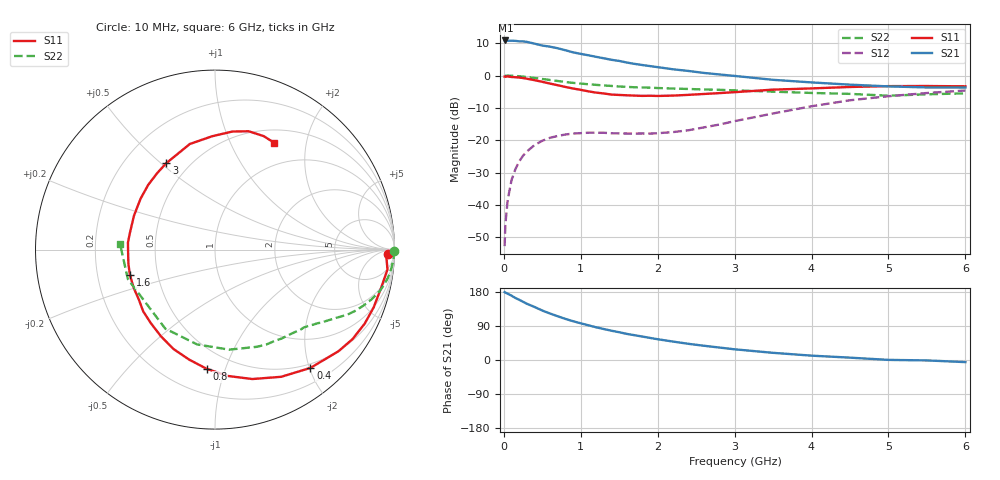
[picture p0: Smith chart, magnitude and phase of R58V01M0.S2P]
! SIEMENS Small Signal Semiconductors
! BFR183
! Si NPN RF Bipolar Junction Transistor in SOT23
! VCE = 8 V  IC = 1 mA
! Common Emitter S-Parameters:  May  1996
# GHz  S  MA  R  50
!  f  S11  S21  S12  S22
! GHz  MAG  ANG  MAG  ANG  MAG  ANG  MAG  ANG
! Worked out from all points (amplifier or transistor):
!   36 points, 10 MHz to 6 GHz, reference 50 ohm
!   highest |S21| = 10.8 dB at 20 MHz (marker M1)
!   |S21| within 3 dB of that: start of sweep to 796.1 MHz
!   unconditionally stable (mu >= 1): 1.684 GHz to 2.971 GHz
!   at 250 MHz: K = 0.15, MSG = 17.7 dB, |S12| = -24.8 dB
!   at 1.4 GHz: K = 0.85, MSG = 11.3 dB, |S12| = -17.8 dB
!   at 6 GHz: K = 0.95, MSG = 0.5 dB, |S12| = -4.6 dB
!   S11 on the Smith chart (normalised r, x): 10 MHz: 39, -23; 400 MHz: 0.43, -2.02; 800 MHz: 0.36, -0.86; 1.6 GHz: 0.34, -0.13; 3 GHz: 0.38, +0.52; 6 GHz: 0.66, +1.48
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0.01  0.9623 -1.3  3.439 179.3  0.0023 89.8  0.9985 -0.4
0.02  0.9561 -2.6  3.483 177.8  0.005 84.9  0.9919 -0.9
0.05  0.9673 -6.6  3.453 174.9  0.0119 83.9  0.997 -2.4
0.1  0.9493 -13.2  3.446 169.8  0.0242 82.0  0.9912 -4.8
0.15  0.9408 -20.0  3.433 163.7  0.0356 77.5  0.9842 -7.3
0.25  0.9144 -33.0  3.369 153.6  0.0576 70.2  0.9626 -11.7
0.3  0.8913 -39.4  3.314 148.3  0.067 67.0  0.9481 -13.9
0.4  0.8469 -51.1  3.106 139.9  0.0842 60.1  0.9157 -17.6
0.5  0.7989 -62.5  2.904 130.5  0.0981 54.2  0.8837 -20.7
0.6  0.7506 -73.9  2.791 122.7  0.1089 49.2  0.8525 -23.6
0.7  0.7077 -84.2  2.639 115.4  0.1164 45.0  0.8227 -26.1
0.8  0.6657 -94.0  2.459 108.5  0.1224 41.0  0.7926 -28.1
0.9  0.6297 -103.2  2.281 102.3  0.1267 38.2  0.7697 -29.8
1.1  0.5691 -122.0  2.053 91.5  0.1305 34.0  0.733 -33.0
1.3  0.5279 -139.2  1.846 81.7  0.1302 31.7  0.7019 -35.8
1.6  0.4944 -163.4  1.586 68.8  0.1268 32.5  0.6671 -39.9
2.2  0.4893 157.3  1.248 48.6  0.1335 44.6  0.6285 -49.2
3  0.5528 119.4  0.985 28.2  0.197 57.4  0.5894 -66.8
3.5  0.6049 103.4  0.858 18.9  0.2591 56.8  0.5629 -82.0
4.5  0.665 81.6  0.722 6.2  0.4144 44.7  0.5202 -122.2
5.5  0.688 66.8  0.654 -1.1  0.5365 27.7  0.5125 -161.3
6  0.6807 61.2  0.653 -5.6  0.5858 17.6  0.5296 176.7
